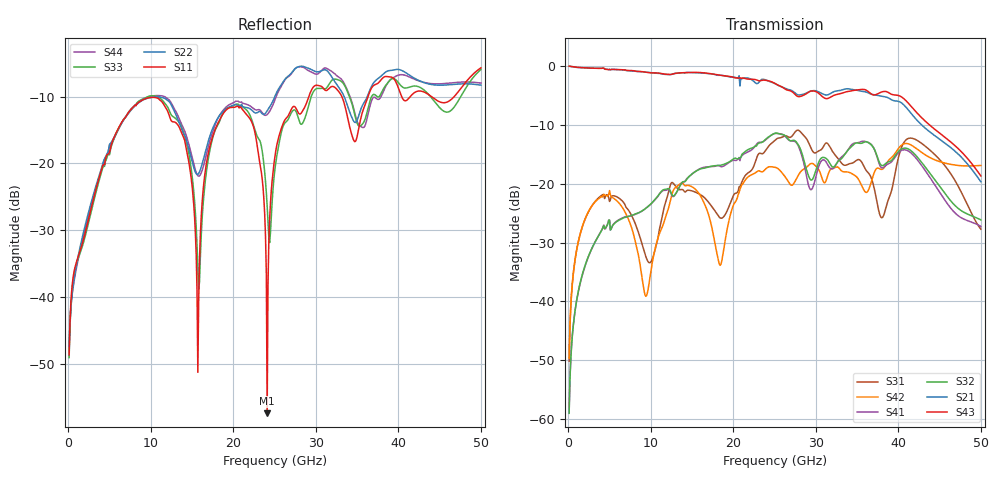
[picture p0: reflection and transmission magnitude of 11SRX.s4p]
! DAC39RF10ACK
! 256-pin FCBGA package
! Texas Instruments 8/20/2022
! Single-ended  S-parameters
! PORT#  PORT_NAME  NET_NAME
! PORT1:  xSRXN.DIEBUMP  xSRXN
! PORT2:  xSRXN.BGA  xSRXN
! PORT3:  xSRXP.DIEBUMP  xSRXP
! PORT4:  xSRXP.BGA  xSRXP
! Touchstone Ver. 1.0
! Number of ports is 4
# Hz	S	MA	R	50.000000
! SCATTERING PARAMETERS  :
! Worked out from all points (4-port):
!   500 points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, 100 MHz to 50 GHz, reference 50 ohm
!   strongest paths, dB at 100 MHz, 12.6 GHz, 25.1 GHz, 37.6 GHz, 50 GHz:
!     S43: 0.0, -1.4, -3.0, -4.6, -18.7
!     S21: 0.0, -1.4, -3.0, -5.0, -19.7
!     S32: -59.0, -22.0, -11.4, -16.0, -26.2
!     S41: -59.0, -22.1, -11.5, -16.3, -27.3
!     S42: -49.6, -21.6, -17.2, -17.4, -16.9
!     S31: -50.2, -19.8, -12.5, -24.5, -27.7
!   lowest |S11| = -57.4 dB at 24.1 GHz (marker M1), VSWR 1.00, Z = 49.9 - j0.0121 ohm
!   |S11| at or under -10 dB: start of sweep to 29.15 GHz; 33.15 GHz to 36.32 GHz (3.173 GHz wide, 9.13 % of centre); 44.01 GHz to 46.76 GHz (2.75 GHz wide, 6.06 % of centre)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
1e8  0.00371 30.4  0.9891 -2.3  0.003097 84.7  0.001134 -95.7
     0.9964 -2.2  0.004283 21.3  0.001025 -98.0  0.003394 72.4
     0.003103 84.6  0.001119 -103.0  0.003532 28.0  0.9888 -2.3
     0.001127 -98.7  0.003303 75.1  0.9966 -2.1  0.004249 22.5
9.7e9  0.3096 -87.7  0.8796 173.1  0.0199 -169.7  0.06427 77.7
       0.883 173.0  0.3087 -107.2  0.06393 78.4  0.013 153.4
       0.02161 -171.4  0.06423 78.9  0.3172 -86.1  0.8789 174.6
       0.06438 77.9  0.01303 156.4  0.8778 174.6  0.3142 -105.9
1.57e10  0.002741 -133.0  0.8776 59.8  0.08478 -52.7  0.132 -33.6
         0.8763 59.8  0.08294 -125.5  0.131 -32.7  0.08572 2.7
         0.08289 -52.7  0.1305 -32.4  0.01661 -159.0  0.8781 62.4
         0.1311 -33.2  0.08507 2.9  0.8818 62.7  0.08093 -134.0
1.8e10  0.1924 -69.7  0.8411 13.6  0.058 -153.3  0.1422 -84.2
        0.8369 13.5  0.212 -98.2  0.1431 -82.1  0.02579 -5.9
        0.05579 -153.6  0.1426 -81.6  0.1886 -69.3  0.8432 16.3
        0.1423 -83.6  0.02581 -5.1  0.8458 16.7  0.2092 -94.6
2.41e10  0.001353 -174.9  0.7525 -106.8  0.1983 -30.5  0.2438 152.2
         0.7525 -106.5  0.2475 -108.7  0.2446 154.8  0.1359 -19.6
         0.2005 -30.5  0.2448 154.3  0.04801 -156.7  0.7557 -102.4
         0.2426 152.2  0.1369 -19.7  0.7529 -102.2  0.2322 -113.9
2.72e10  0.2644 -74.1  0.6129 -167.0  0.2587 -159.2  0.2311 60.0
         0.6116 -166.8  0.4886 -118.4  0.2319 65.1  0.09828 -145.2
         0.258 -158.7  0.2335 65.0  0.2476 -80.2  0.6014 -162.6
         0.2305 59.6  0.09791 -145.5  0.5989 -162.8  0.4851 -118.2
5e10  0.5188 -103.7  0.09948 124.7  0.04115 148.0  0.05336 8.2
      0.1038 128.6  0.3856 -169.0  0.04776 19.9  0.1364 22.5
      0.04106 148.7  0.04925 13.1  0.5039 -98.3  0.1125 133.3
      0.04332 15.0  0.1428 16.7  0.1163 132.6  0.3994 -166.4
